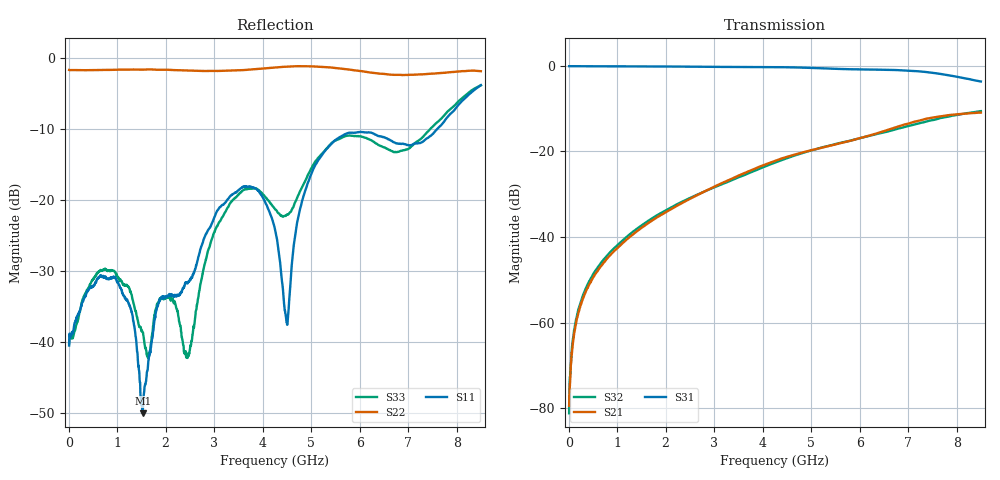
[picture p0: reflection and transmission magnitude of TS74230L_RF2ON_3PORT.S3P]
!Agilent Technologies,E5071C,MY46522130,B.12.04
!Date: Wed Jul 30 10:25:27 2025
!Data & Calibration Information:
!Freq	S11:SOLT3(ON)	S13:SOLT3(ON)	S14:SOLT3(ON)
!	S31:SOLT3(ON)	S33:SOLT3(ON)	S34:SOLT3(ON)
!	S41:SOLT3(ON)	S43:SOLT3(ON)	S44:SOLT3(ON)
!PortZ  Port1:50+j0  Port3:50+j0  Port4:50+j0
!Above PortZ is port z conversion or system Z0 setting when saving the data.
!When reading, reference impedance value at option line is always used.
# Hz S dB R 50
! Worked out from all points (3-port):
!   1601 points, 10 MHz to 8.5 GHz, reference 50 ohm
!   strongest paths, dB at 10 MHz, 2.132 GHz, 4.255 GHz, 6.378 GHz, 8.5 GHz:
!     S31: -0.1, -0.2, -0.4, -0.9, -3.7
!     S21: -79.5, -33.4, -22.2, -15.7, -11.0
!     S32: -81.2, -33.0, -22.6, -15.9, -10.6
!   lowest |S11| = -50.0 dB at 1.528 GHz (marker M1), VSWR 1.01, Z = 49.7 + j0.1 ohm
!   |S11| at or under -10 dB: start of sweep to 7.603 GHz
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1e7  -40.51 25.6  -79.53 35.8  -0.13 -0.3
     -79.45 39.8  -1.72 179.4  -79.64 44.5
     -0.13 -0.3  -81.21 45.3  -40.21 24.1
3.602125e8  -33.28 56.1  -52.62 93.5  -0.15 -6.2
            -52.54 93.4  -1.75 171.1  -51.85 91.3
            -0.15 -6.2  -51.93 91.8  -33.04 53.8
1.002269e9  -31.61 75.4  -42.63 101.9  -0.18 -17.0
            -42.67 102.0  -1.68 156.2  -41.99 95.7
            -0.18 -17.0  -41.98 95.9  -30.77 46.9
1.527588e9  -50.05 161.3  -37.69 104.4  -0.19 -25.9
            -37.69 104.4  -1.68 145.1  -37.14 95.5
            -0.19 -25.9  -37.13 95.4  -38.62 -22.7
2.461488e9  -31.55 -50.5  -31.36 102.1  -0.24 -41.9
            -31.36 101.9  -1.80 125.2  -31.15 88.0
            -0.24 -41.9  -31.13 88.1  -41.79 -43.7
3.092931e9  -21.24 -7.6  -27.77 97.5  -0.30 -52.9
            -27.79 97.2  -1.86 110.5  -28.00 81.5
            -0.30 -53.0  -28.01 81.7  -23.29 42.6
4.255e9  -24.15 -8.2  -22.27 80.8  -0.36 -73.8
         -22.25 80.5  -1.38 87.0  -22.68 65.9
         -0.37 -73.8  -22.65 66.2  -21.31 58.7
4.493781e9  -37.21 -96.9  -21.30 76.0  -0.38 -78.4
            -21.35 75.7  -1.25 84.1  -21.63 61.2
            -0.39 -78.5  -21.65 61.6  -22.14 100.2
5.289719e9  -13.09 176.9  -19.01 61.7  -0.64 -93.9
            -18.97 61.2  -1.32 76.3  -18.90 44.7
            -0.65 -94.0  -18.93 44.5  -13.01 151.1
8.5e9  -3.86 105.9  -11.03 -8.7  -3.72 -160.5
       -10.98 -8.9  -1.89 30.4  -10.67 -26.1
       -3.71 -160.7  -10.63 -25.3  -3.88 80.9
